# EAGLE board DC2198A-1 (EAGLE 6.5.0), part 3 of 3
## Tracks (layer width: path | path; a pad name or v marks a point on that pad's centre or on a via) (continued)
VSNSP_CH12 (continued)
  Top 0.165: U10.B10 63.25,19.25 63.25,14.38 63,14.12 61.88,14.12 | 61.88,14.12 | 61.88,14.12 VSNSN23.1
  Bottom 0.203: 63.5,12.45 R88.2 | C58.2 61.85,12.45
  Bottom 0.406: VSNSN23.1 61.85,12.45 63.5,12.45
VSNSP_CH13  (via drill 0.25)
  Top 0.165: U10.C8 62.25,22.25 66.62,22.25 66.88,22.5 71.62,22.5 v71.62,22.62
  Bottom 0.165: v71.62,22.62 71.62,15 72,14.62 72.88,14.62 72.88,14.63 VSNSN21.1
  Bottom 0.203: 75.06,12.45 R86.2 | C57.2 73.41,12.45
  Bottom 0.406: VSNSN21.1 73.41,12.45 75.06,12.45
VSNSP_CH14  (via drill 0.25)
  Top 0.165: U10.E8 v60.25,21.25 | v70.38,21.62 70.5,21.75 71.5,21.75 71.62,21.62 71.62,20.38 71.88,20.12 82,20.12 82.38,20.5 83.38,20.5 83.5,20.38 v83.5,20
  Route15 0.165: v60.25,21.25 70.25,21.25 70.38,21.38 v70.38,21.62
  Bottom 0.165: v83.5,20 83.5,15.12 83.75,14.88 84.75,14.88 84.94,14.69 84.94,14.12 VSNSN19.1
  Bottom 0.203: 86.61,12.45 R84.2 | 84.96,12.45 C56.2
  Bottom 0.406: VSNSN19.1 84.96,12.45 86.61,12.45
VSNSP_CH15  (via drill 0.25)
  Top 0.165: U10.A8 66.75,21.75 67.12,22.12 71.62,22.12 72,21.75 72,20.62 72.12,20.5 81.75,20.5 82.12,20.88 84,20.88 84.38,20.5 93.25,20.5 93.88,21.12 v96.5,21.12
  Bottom 0.165: v96.5,21.12 96.5,14.12 VSNSN17.1
  Bottom 0.203: 98.17,12.45 R82.2 | 96.52,12.45 C55.2
  Bottom 0.406: VSNSN17.1 96.52,12.45 98.17,12.45

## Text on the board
tPlace: CH0 1.0V | CH1 1.1V | CH2 1.2V | CH3 1.3V | CH4 1.4V | CH5 1.5V | CH6 1.7V | CH7 1.8V | GND | INSTALL CONNECTORS | ON TOP SIDE | F | E | M | A | L | E | GND | 6-14V | 0.3A | 0.3A | 0.3A | 0.3A | 0.3A | 0.3A | 0.3A | 0.3A | SCL | - | + | SHARE_CLK | CONTROL | A1 | SDA | LTC2980CY | FAULT | ALERT | DEMO CIRCUIT 2198A | LTC2980CY | + | 16-CHANNEL | ALERT | GND | GND | GND | GND | POWER SYSTEM | MANAGER | +5V | FAULT | RESET | CREATE FAULT | RUN | OFF | CONTROL | 0.3A | 0.3A | 0.3A | 0.3A | 0.3A | 0.3A | 0.3A | 0.3A | M | A | L | E | RESET | CH8 2.0V | CH9 2.2V | CH10 2.5V | CH11 2.7V | CH12 3.0V | CH13 3.1V | CH14 3.2V | CH15 3.3V
bPlace: CH0 1.0V | CH1 1.1V | CH2 1.2V | CH3 1.3V | CH4 1.4V | CH5 1.5V | CH6 1.7V | CH7 1.8V | REV 1 | RUN | VS | DAC | RUN | VS | DAC | RUN | VS | DAC | RUN | VS | DAC | RUN | VS | DAC | RUN | VS | DAC | RUN | VS | DAC | RUN | VS | DAC | LTC CONFIDENTIAL - FOR CUSTOMER USE ONLY | DAC | VS | RUN | DAC | VS | RUN | DAC | VS | RUN | DAC | VS | RUN | DAC | VS | RUN | DAC | VS | RUN | DAC | VS | RUN | DAC | VS | RUN | OPEN | A2 | A1 | MUX | SCLK | A0 | 1 | CH8 2.0V | CH9 2.2V | CH10 2.5V | CH11 2.7V | CH12 3.0V | CH13 3.1V | CH14 3.2V | CH15 3.3V
tStop: KVL | LTC2980CY | 16-CHANNEL | POWER MANAGER | (408) 432-1900 | www.linear.com
bStop: POWER MANAGER | 16-CHANNEL | LTC2980CY | (408) 432-1900 | www.linear.com
d_FabDrawing: DRILL TABLE | 1.825" | 0.00" | 5.185" | 0.00" | SHOWN FROM TOP SIDE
